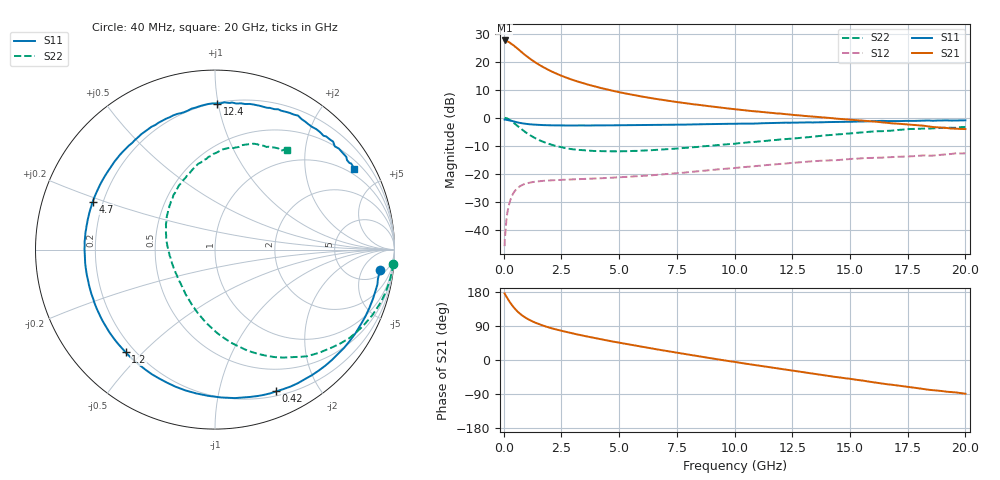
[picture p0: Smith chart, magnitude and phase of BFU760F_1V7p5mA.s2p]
! Filename:  P:\Prog\Test\Noise\ATS_data\Testdata_Net\Split files Spar\BFU760F_2W_C1_1V_5mA_60mA_Bias2_D.s2p
! Date/Time: Mon 06/Feb/2012 15:06:00
! BFU760_2W_C1_1V_5mA_60mA_Bias2_R.s2p
! MDIF S-parameter v. bias file
! BFU760_2W_C1_1V_5mA_60mA
! Date/time Fri Mar 18 10:56:44 2011
! VAR V_out= 1.0001
! VAR I_out= 7.5200
! VAR V_in= 0.7694
! VAR I_in= 0.0217
! Device data file deembeded for feedlines and parallel
! Original file: \Split files Spar\BFU760_2W_C1_1V_5mA_60mA_Bias2_R.s2p
! Feed-files: PR003V01_101208_Feed1.s2p, PR003V01_101208_Feed2.s2p
! Parallel-file: PR003V01_101208_Par.s2p
# MHz S MA R 50
!  Freq-MHz  S11-mag  S11-arg  S21-mag  S21-arg  S12-mag  S12-arg  S22-mag  S22-arg
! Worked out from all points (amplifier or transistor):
!   167 points, 40 MHz to 20 GHz, reference 50 ohm
!   highest |S21| = 27.6 dB at 40 MHz (marker M1)
!   |S21| within 3 dB of that: start of sweep to 611.4 MHz
!   unconditionally stable (mu >= 1): 5.573 GHz to 13.95 GHz; 14.58738 GHz to 14.60718 GHz
!   at 550 MHz: K = 0.10, MSG = 25.3 dB, |S12| = -25.5 dB
!   at 4.2 GHz: K = 0.82, MSG = 16.1 dB, |S12| = -21.6 dB
!   at 20 GHz: K = 0.85, MSG = 4.3 dB, |S12| = -12.7 dB
!   S11 on the Smith chart (normalised r, x): 40 MHz: 7, -12; 420 MHz: 0.25, -1.49; 1.2 GHz: 0.17, -0.44; 4.7 GHz: 0.16, +0.18; 12.4 GHz: 0.21, +0.99; 20 GHz: 0.76, +3.56
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40  0.9268 -7.0  23.92 175.8  0.005092 86.2  0.9953 -4.6
50  0.9228 -9.3  23.92 174.2  0.006659 81.5  0.9941 -5.8
60  0.9223 -10.2  23.59 173.3  0.007544 83.6  0.9937 -6.9
140  0.917 -24.0  23.28 165.0  0.01769 77.5  0.9735 -16.2
240  0.8986 -40.5  22.25 155.0  0.02905 68.8  0.9291 -27.0
340  0.8783 -55.3  20.73 146.2  0.03862 61.0  0.8708 -37.1
420  0.8603 -66.6  19.73 139.8  0.04502 55.7  0.8213 -44.0
600  0.8243 -87.8  17.1 127.9  0.05542 45.5  0.7112 -57.8
800  0.7949 -106.0  14.53 117.6  0.06283 37.5  0.6107 -69.7
1000  0.7733 -120.0  12.45 109.7  0.06737 31.9  0.5317 -79.5
1200  0.7584 -131.1  10.84 103.2  0.07037 27.7  0.4712 -87.6
1550  0.743 -145.6  8.739 94.2  0.07356 22.6  0.3961 -99.3
1950  0.7321 -157.8  7.102 86.0  0.07568 18.9  0.3418 -110.5
2500  0.7278 -170.1  5.609 77.1  0.0776 16.0  0.2974 -123.5
3400  0.727 175.1  4.181 64.7  0.08043 13.3  0.2641 -140.1
4700  0.7317 158.5  3.042 49.0  0.08495 12.1  0.2511 -160.7
6800  0.7455 136.9  2.102 26.4  0.09665 10.8  0.2695 172.9
10200  0.7834 107.2  1.39 -7.0  0.1288 3.4  0.3512 136.3
12400  0.8137 89.2  1.14 -27.0  0.1549 -5.7  0.4209 115.5
13400  0.8224 81.6  1.046 -35.8  0.1668 -11.7  0.4582 106.7
16800  0.8725 55.0  0.7945 -65.2  0.1978 -31.6  0.5873 76.9
20000  0.8982 30.1  0.6267 -89.0  0.2307 -53.0  0.6841 54.1
